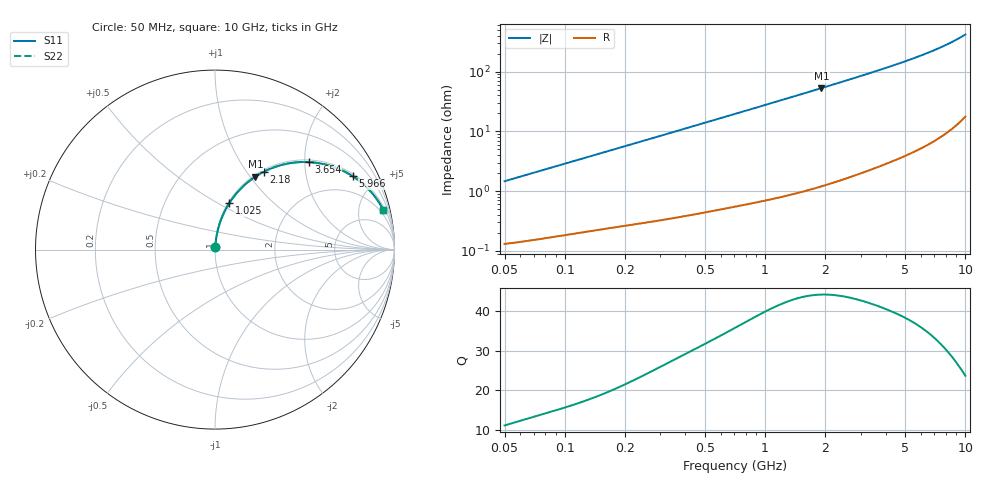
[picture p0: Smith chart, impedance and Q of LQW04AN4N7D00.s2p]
!Murata Part Number: LQW04AN4N7D00
!These Parameters are Measured in Series Mode Connection
!  o--[Z]--o
!Port1  Port2
!  o-------o
!Freq. Start=50[MHz] Stop=10[GHz], 401[Steps]
# Hz S RI R 50
!Freq.(Hz)	S 11(Real)	S 11(Imag)	S 21(Real)	S 21(Imag)	S 12(Real)	S 12(Imag)	S 22(Real)	S 22(Imag)
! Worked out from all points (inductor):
!   401 points, 50 MHz to 10 GHz, reference 50 ohm
!   read as one part in series: L = 4.63 nH near 51.34 MHz
!   highest Q = 44.2 at 1.91 GHz (marker M1), where L = 4.42 nH
!   S11 on the Smith chart (normalised r, x): 50 MHz: 1.00, +0.03; 1.025 GHz: 1.01, +0.57; 2.18 GHz: 1.03, +1.21; 3.654 GHz: 1.05, +2.09; 5.966 GHz: 1.10, +3.70; 10 GHz: 1.35, +8.39
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5e7  0.00152 0.0146  0.9985 -0.0146  0.9985 -0.0146  0.00152 0.0146
1.214486e8  0.00323 0.0346  0.9968 -0.0346  0.9968 -0.0346  0.00323 0.0346
1.956524e8  0.00563 0.0549  0.9944 -0.0549  0.9944 -0.0549  0.00563 0.0549
2.949953e8  0.00996 0.0818  0.99 -0.0818  0.99 -0.0818  0.00996 0.0818
4.689809e8  0.0208 0.1276  0.9792 -0.1276  0.9792 -0.1276  0.0208 0.1276
7.071068e8  0.042 0.187  0.958 -0.187  0.958 -0.187  0.042 0.187
1.024606e9  0.08 0.2592  0.92 -0.2592  0.92 -0.2592  0.08 0.2592
1.335391e9  0.126 0.3204  0.874 -0.3204  0.874 -0.3204  0.126 0.3204
1.717543e9  0.1905 0.3815  0.8095 -0.3815  0.8095 -0.3815  0.1905 0.3815
1.909537e9  0.2248 0.4063  0.7752 -0.4063  0.7752 -0.4063  0.2248 0.4063
2.179987e9  0.274 0.4348  0.726 -0.4348  0.726 -0.4348  0.274 0.4348
2.879108e9  0.3986 0.4781  0.6014 -0.4781  0.6014 -0.4781  0.3986 0.4781
3.243629e9  0.4589 0.4866  0.5411 -0.4866  0.5411 -0.4866  0.4589 0.4866
3.654301e9  0.5216 0.4876  0.4784 -0.4876  0.4784 -0.4876  0.5216 0.4876
4.171863e9  0.5919 0.4792  0.4081 -0.4792  0.4081 -0.4792  0.5919 0.4792
4.955797e9  0.6806 0.4534  0.3194 -0.4534  0.3194 -0.4534  0.6806 0.4534
5.965537e9  0.768 0.4085  0.232 -0.4085  0.232 -0.4085  0.768 0.4085
6.810442e9  0.8228 0.3674  0.1772 -0.3674  0.1772 -0.3674  0.8228 0.3674
7.775012e9  0.8701 0.3205  0.1299 -0.3205  0.1299 -0.3205  0.8701 0.3205
8.644138e9  0.9022 0.2799  0.0978 -0.2799  0.0978 -0.2799  0.9022 0.2799
9.738562e9  0.9322 0.2318  0.0678 -0.2318  0.0678 -0.2318  0.9322 0.2318
1e10  0.938 0.2209  0.062 -0.2209  0.062 -0.2209  0.938 0.2209
